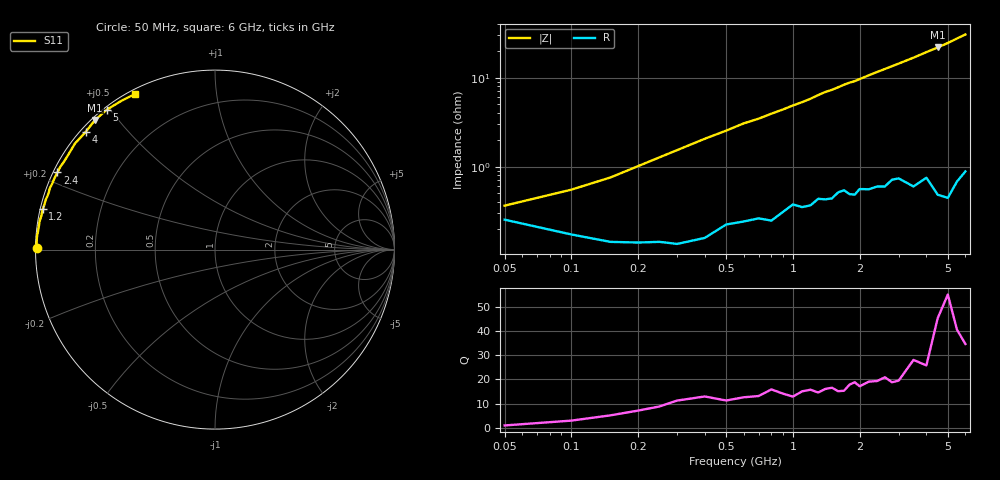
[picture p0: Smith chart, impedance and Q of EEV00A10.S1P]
! Infineon Technologies  Discrete & RF Semiconductors
! BBY55-02W
! Si Tuning Diode in SCD-80
! VR =
! S-Parameters:  June  2000
# GHz  S  MA  R  50
!  f  S11
! GHz  MAG  ANG
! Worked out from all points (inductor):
!   34 points, 50 MHz to 6 GHz, reference 50 ohm
!   read as one part to ground: L = 799 pH near 100 MHz
!   highest Q = 45.2 at 4.5 GHz (marker M1), where L = 773 pH
!   S11 on the Smith chart (normalised r, x): 50 MHz: 0.01, +0.01; 1.2 GHz: 0.01, +0.12; 2.4 GHz: 0.01, +0.23; 4 GHz: 0.02, +0.39; 5 GHz: 0.01, +0.49; 6 GHz: 0.02, +0.61
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0.05  0.9899 179.4
0.1  0.9931 178.8
0.15  0.9943 178.3
0.3  0.9946 176.5
0.6  0.9904 173.0
0.7  0.9896 172.1
0.8  0.9902 171.0
1  0.9852 168.9
1.1  0.9862 167.9
1.2  0.9856 166.8
1.3  0.983 165.5
1.4  0.9833 164.3
1.5  0.9829 163.4
1.6  0.9801 162.3
1.7  0.9791 161.1
1.8  0.9811 160.1
1.9  0.9814 159.3
2  0.9786 158.2
2.2  0.9789 156.0
2.4  0.9775 153.9
2.6  0.9777 151.9
3  0.9731 147.9
3.5  0.9787 142.9
4  0.9742 137.7
4.5  0.9839 132.8
5  0.9857 127.7
5.5  0.9793 122.3
6  0.9746 117.1
